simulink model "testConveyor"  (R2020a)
settings: Solver=FixedStepDiscrete  StartTime=0.0  StopTime=20.1  RelTol=1e-3  EnableMultiTasking=on

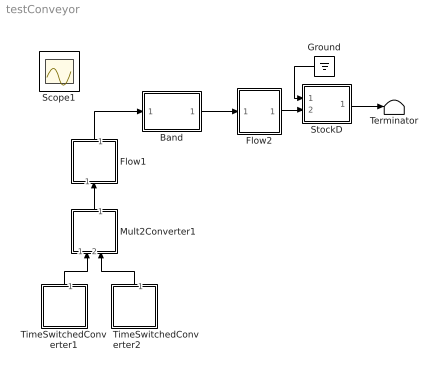
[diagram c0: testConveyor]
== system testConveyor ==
  Band : Subsystem  mask{ndelay=3, dt=1, t0=0.1}
      mask prompts: ndelay "Transit time"; dt "Sample Period"; t0 "Start Time"
  Flow1 : Subsystem
  Flow2 : Subsystem
  Ground : Ground
  Mult2Converter1 : Subsystem
  StockD : Subsystem  mask{m0=0, dt=1, t0=0.1}
      mask prompts: m0 "Initial Value"; dt "Sample Period"; t0 "Start Time"
  Terminator : Terminator
  TimeSwitchedConverter1 : Subsystem  mask{t0=3, oldval=0, newval=1}
      mask prompts: t0 "switchTime"; oldval "oldValue"; newval "newValue"
  TimeSwitchedConverter2 : Subsystem  mask{t0=13, oldval=5, newval=0}
      mask prompts: t0 "switchTime"; oldval "oldValue"; newval "newValue"
  Scope1 : Scope
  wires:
  Flow1/1(Out1) -> Band/1(In)
  Mult2Converter1/1(Out1) -> Flow1/1(In1)
  TimeSwitchedConverter1/1(Out1) -> Mult2Converter1/1(In1)
  TimeSwitchedConverter2/1(Out1) -> Mult2Converter1/2(In2)
  Band/1(Out) -> Flow2/1(In1)
  Flow2/1(Out1) -> StockD/2(In2)
  StockD/1(Out1) -> Terminator/1
  Ground/1 -> StockD/1(In1)

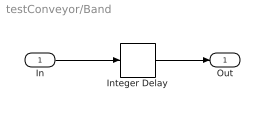
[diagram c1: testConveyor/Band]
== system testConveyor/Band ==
  In : Inport
  Integer Delay : Delay  DelayLength=ndelay  SampleTime=[dt,t0]
  Out : Outport
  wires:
  In/1 -> Integer Delay/1
  Integer Delay/1 -> Out/1

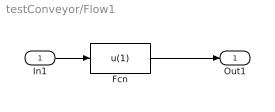
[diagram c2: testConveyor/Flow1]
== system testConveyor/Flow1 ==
  In1 : Inport
  Fcn : Fcn  Expr=u(1)
  Out1 : Outport
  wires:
  Fcn/1 -> Out1/1
  In1/1 -> Fcn/1

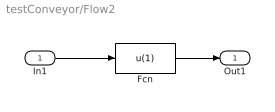
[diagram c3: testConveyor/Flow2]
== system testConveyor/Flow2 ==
  In1 : Inport
  Fcn : Fcn  Expr=u(1)
  Out1 : Outport
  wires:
  Fcn/1 -> Out1/1
  In1/1 -> Fcn/1

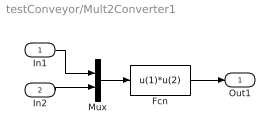
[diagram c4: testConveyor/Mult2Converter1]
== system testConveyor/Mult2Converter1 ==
  In1 : Inport
  In2 : Inport  Port=2
  Fcn : Fcn  Expr=u(1)*u(2)
  Mux : Mux  Inputs=2
  Out1 : Outport
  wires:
  Fcn/1 -> Out1/1
  Mux/1 -> Fcn/1
  In1/1 -> Mux/1
  In2/1 -> Mux/2

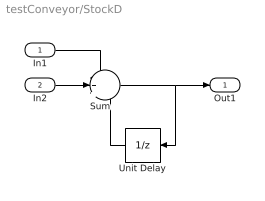
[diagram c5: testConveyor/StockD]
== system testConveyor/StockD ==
  In1 : Inport
  In2 : Inport  Port=2
  Sum : Sum  Inputs=-++  SaturateOnIntegerOverflow=on
  Unit Delay : UnitDelay  InitialCondition=m0  SampleTime=[dt, t0]  HasFrameUpgradeWarning=on
  Out1 : Outport
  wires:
  In1/1 -> Sum/1
  Sum/1 -> Out1/1, Unit Delay/1
  In2/1 -> Sum/2
  Unit Delay/1 -> Sum/3

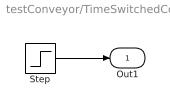
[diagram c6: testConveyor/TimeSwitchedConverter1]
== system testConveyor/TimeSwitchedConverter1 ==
  Step : Step  Time=t0  Before=oldval  After=newval
  Out1 : Outport
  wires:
  Step/1 -> Out1/1

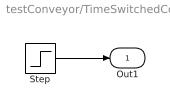
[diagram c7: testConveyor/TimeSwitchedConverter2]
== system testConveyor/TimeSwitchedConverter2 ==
  Step : Step  Time=t0  Before=oldval  After=newval
  Out1 : Outport
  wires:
  Step/1 -> Out1/1
